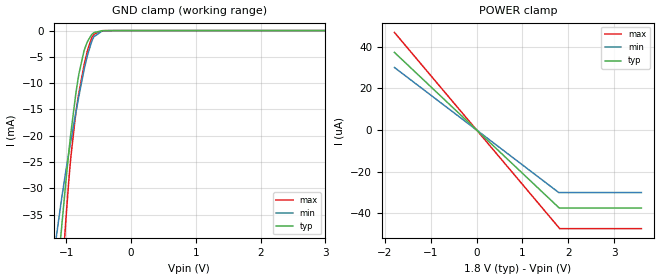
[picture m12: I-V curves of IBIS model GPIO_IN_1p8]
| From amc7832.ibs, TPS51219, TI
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|   Model
[Model]   GPIO_IN_1p8
Model_type   Input
Vinl = 0.45
Vinh = 1.26
|   typ   min   max
C_comp   1pF   1pF   1pF
[Voltage Range]   1.8   1.79   1.81
[Temperature Range]   27   125   -40
[Power Clamp Reference]   1.8   1.79   1.81
[GND Clamp Reference]   -0   -0   -0
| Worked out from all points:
|   GND clamp passes 1 mA (typ) near -0.62 V on its own axis
[GND Clamp]
|   Voltage   I(typ)   I(min)   I(max)
-1.795V   -152mA     -104.8mA   -207mA
-1.233V   -60.35mA   -46.12mA   -81.02mA
-1.087V   -39.15mA   -33.05mA   -50.69mA
-1.076V   -37.66mA   -32.13mA   -48.56mA
-1.012V   -29.05mA   -26.87mA   -36.43mA
-930.6mV  -19.36mA   -20.88mA   -23.89mA
-828mV    -9.753mA   -13.8mA    -13.36mA
-714.6mV  -3.357mA   -6.743mA   -5.845mA
-671.4mV  -1.997mA   -4.526mA   -3.637mA
-574.2mV  -388.6uA   -1.157mA   -676.9uA
-352.8mV  -8.303uA   -16.19uA   -9.726uA
3.595V    0A         0A         0A
[POWER Clamp]
|   Voltage   I(typ)   I(min)   I(max)
-1.795V   37.36uA    30.1uA     46.98uA
1.791V    -37.33uA   -30.1uA    -46.92uA
1.813V    -37.56uA   -30.1uA    -47.49uA
3.595V    -37.56uA   -30.1uA    -47.49uA
